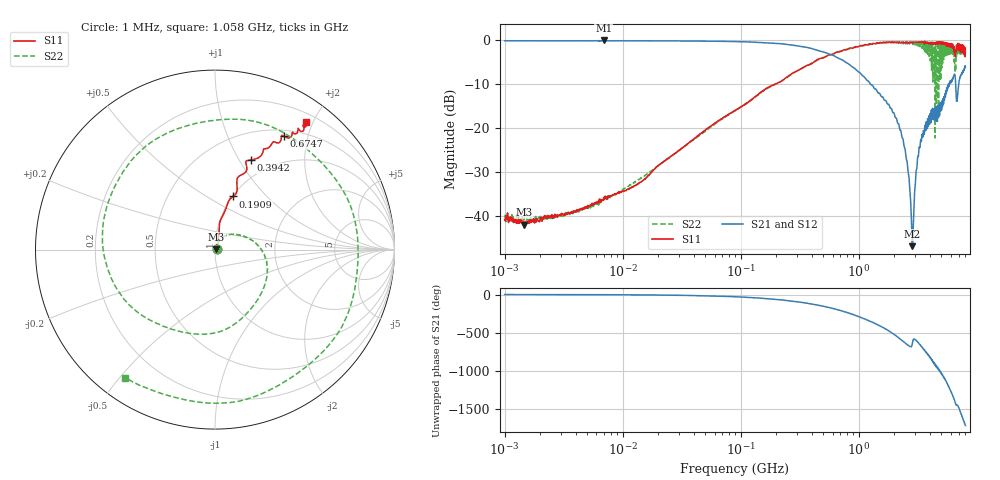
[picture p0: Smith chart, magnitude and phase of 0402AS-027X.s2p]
!s-Parameter Generated by FASTRON Sdn. Bhd.
!FASTRON P/N : 0402AS-027X
!Keysight Technologies: E5071C_MY46733604_B.14.02
!Date: Mon Dec 01 10:33:54 2025
!Version  :Rev00  Mon Dec 01 10:33:54 2025
!Data & Calibration Information:
!Freq  S11:SOLT2(ON)  S21:SOLT2(ON)  S12:SOLT2(ON)  S22:SOLT2(ON)
!PortZ  Port1:50+j0  Port2:50+j0
!When reading reference impedance value at option line is always used.
! Remarks : This data is being provided solely for informational purposes.
# Hz S dB R 50
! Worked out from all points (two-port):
!   1601 points, 1 MHz to 8 GHz, reference 50 ohm
!   highest |S21| = -0.01 dB at 6.912 MHz (marker M1); lowest = -47.0 dB at 2.839 GHz (marker M2)
!   |S21| within 3 dB of the highest: start of sweep to 548.9 MHz
!   lowest |S11| = -42.1 dB at 1.45 MHz (marker M3), VSWR 1.02, Z = 50.7 + j0.254 ohm
!   |S11| at or under -10 dB: start of sweep to 195.4 MHz
!   |S22| runs from -41.7 to -0.1 dB; largest |S21 - S12| = 0.015
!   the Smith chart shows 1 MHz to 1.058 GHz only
!   S11 on the Smith chart (normalised r, x): 1 MHz: 1.02, +0.01; 190.9 MHz: 1.00, +0.66; 394.2 MHz: 0.80, +1.13; 674.7 MHz: 0.58, +1.62; 1.058 GHz: 0.33, +1.90
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1000000  -40.90 16.5  -0.09 -0.3  -0.07 -0.4  -39.90 14.0
1450094  -42.10 18.6  -0.08 -0.5  -0.08 -0.5  -41.00 9.9
4479405  -38.50 42.7  -0.09 -1.5  -0.08 -1.6  -38.70 43.1
6911657  -35.90 44.6  -0.01 -2.5  -0.04 -2.2  -35.90 45.6
2.00676e7  -28.60 68.5  -0.10 -6.7  -0.10 -6.6  -28.50 65.4
8.994653e7  -16.00 79.8  -0.26 -29.3  -0.26 -29.2  -16.00 30.7
1.90914e8  -10.10 71.5  -0.64 -60.8  -0.64 -60.8  -10.20 -19.6
3.942396e8  -5.37 68.1  -1.81 -123.0  -1.80 -123.0  -5.27 -137.0
4.006501e8  -5.28 67.1  -1.86 -125.0  -1.85 -125.0  -5.16 -140.0
6.746764e8  -2.62 58.7  -4.08 158.0  -4.07 157.0  -2.56 74.9
8.418203e8  -1.74 55.6  -5.61 112.0  -5.60 112.0  -1.87 -13.7
1.058419e9  -1.21 54.5  -7.86 56.3  -7.86 56.1  -1.20 -125.0
1.349549e9  -0.71 58.7  -10.90 -13.4  -10.90 -13.5  -0.73 90.6
1.550632e9  -0.54 63.7  -12.80 -59.1  -12.80 -59.3  -0.51 -5.9
1.7949e9  -0.39 69.3  -14.60 -116.0  -14.60 -116.0  -0.55 -125.0
2.071864e9  -0.45 74.9  -17.70 179.0  -17.70 179.0  -0.52 99.2
2.44288e9  -0.56 80.4  -24.50 93.5  -24.50 93.5  -0.38 -82.2
2.839031e9  -0.54 91.0  -47.00 76.2  -47.00 76.7  -0.42 90.6
3.183204e9  -0.37 99.5  -26.50 89.2  -26.50 88.8  -0.79 -94.9
3.548043e9  -0.40 110.0  -20.80 -0.2  -20.70 -0.8  -2.11 74.7
3.912882e9  -0.75 115.0  -17.60 -73.8  -17.60 -74.3  -0.58 -72.0
8e9  -1.73 -113.0  -6.08 86.6  -6.08 86.2  -3.64 123.0
